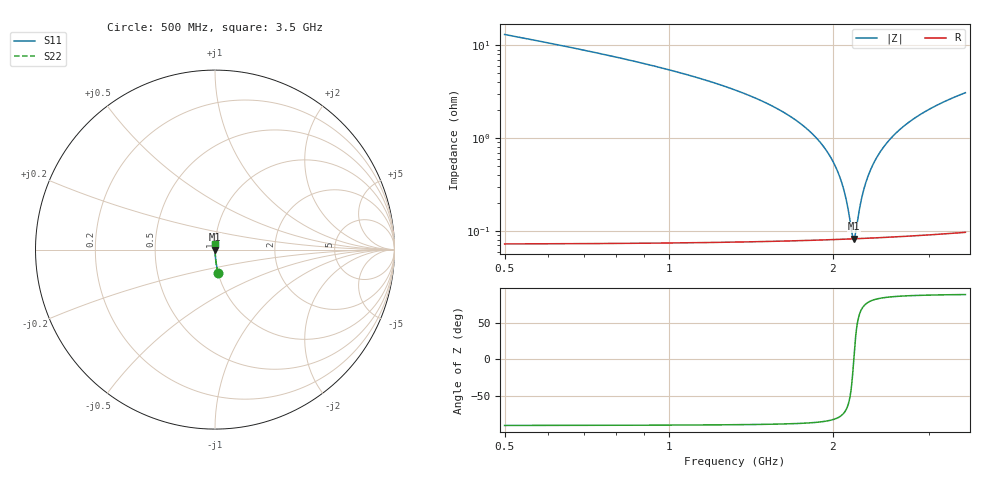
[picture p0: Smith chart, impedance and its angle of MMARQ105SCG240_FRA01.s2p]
! MMARQ105SCG240_FRA01  S-PARAMETER MODEL  ( General Type )
! Model Generated by TAIYO YUDEN Corporation (http://www.ty-top.com)
! Version 1.0
! TAIYO YUDEN Control No. 200326
! Copyright(c) 2020 TAIYO YUDEN CO.,LTD. All Rights Reserved.
! Product Description (link to TY-COMPAS)
! https://ds.yuden.co.jp/TYCOMPAS/or/detail?pn=MMARQ105SCG240JFRA01&u=M
! Products Name : Multilayer Ceramic Capacitors
! Characteristics :
!  Capacitance : 24 pF , Rated Voltage : 250V , TCC : CG / C0G
!  Case Size : 1.0 x 0.5 / 0.039 x 0.02 [mm/inch] , Thickness : 0.5 / 0.02 [mm/inch]
!  (Conditions: Temperature = 25 degC , DC Bias Current/Voltage = 0A / 0V)
! External Node Assignments :
!  1  o---| |---o  2
! GND o---------o GND
! Frequency Range : 500MHz  -  3.5GHz  [ 401 STEP ]
# MHz S RI R 50
! Freq[MHz].  S11 Real  S11 Imag  S21 Real  S21 Imag  S12 Real  S12 Imag  S22 Real  S22 Imag
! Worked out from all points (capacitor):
!   401 points, 500 MHz to 3.5 GHz, reference 50 ohm
!   read as one part in series: C = 23 pF near 515 MHz
!   lowest |Z| = 83 mohm at 2.188 GHz (marker M1)
!   series resonance near 2.184 GHz, so ESL is about 230 pH
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500  0.0176 -0.1287  0.9824 0.1287  0.9824 0.1287  0.0176 -0.1287
1002.5  0.00369 -0.0542  0.9963 0.0542  0.9963 0.0542  0.00369 -0.0542
1505  0.00135 -0.0241  0.9986 0.0241  0.9986 0.0241  0.00135 -0.0241
1670  0.00108 -0.0172  0.9989 0.0172  0.9989 0.0172  0.00108 -0.0172
1805  0.00094 -0.0121  0.9991 0.0121  0.9991 0.0121  0.00094 -0.0121
1917.5  0.00087 -0.00826  0.9991 0.00826  0.9991 0.00826  0.00087 -0.00826
2000  0.00084 -0.00558  0.9992 0.00558  0.9992 0.00558  0.00084 -0.00558
2052.5  0.000829 -0.00394  0.9992 0.00394  0.9992 0.00394  0.000829 -0.00394
2090  0.000824 -0.00279  0.9992 0.00279  0.9992 0.00279  0.000824 -0.00279
2127.5  0.000822 -0.00167  0.9992 0.00167  0.9992 0.00167  0.000822 -0.00167
2165  0.000823 -0.000566  0.9992 0.000566  0.9992 0.000566  0.000823 -0.000566
2180  0.000824 -0.00013  0.9992 0.00013  0.9992 0.00013  0.000824 -0.00013
2187.5  0.000825 8.68e-05  0.9992 -8.68e-05  0.9992 -8.68e-05  0.000825 8.68e-05
2202.5  0.000827 0.000519  0.9992 -0.000519  0.9992 -0.000519  0.000827 0.000519
2240  0.000832 0.00159  0.9992 -0.00159  0.9992 -0.00159  0.000832 0.00159
2262.5  0.000837 0.00222  0.9992 -0.00222  0.9992 -0.00222  0.000837 0.00222
2315  0.00085 0.00367  0.9991 -0.00367  0.9991 -0.00367  0.00085 0.00367
2397.5  0.000879 0.00589  0.9991 -0.00589  0.9991 -0.00589  0.000879 0.00589
2502.5  0.000929 0.00861  0.9991 -0.00861  0.9991 -0.00861  0.000929 0.00861
2712.5  0.00107 0.0138  0.9989 -0.0138  0.9989 -0.0138  0.00107 0.0138
3005  0.00133 0.0205  0.9987 -0.0205  0.9987 -0.0205  0.00133 0.0205
3500  0.00192 0.0308  0.9981 -0.0308  0.9981 -0.0308  0.00192 0.0308
